TYPE APCControlDI :
STRUCT
	P1ZeroOffsetOutRangeAlm_b	:	BOOL	;
	P1ZeroAdjOutRangeAlm_b	:	BOOL	;
	P1SpanAdjOutRangeAlm_b	:	BOOL	;
	P2ZeroOffsetOutRangeAlm_b	:	BOOL	;
	P2ZeroAdjOutRangeAlm_b	:	BOOL	;
	P2SpanAdjOutRangeAlm_b	:	BOOL	;
	P1PressCtrlInterlockAlm_b	:	BOOL	;
	P2PressCtrlInterlockAlm_b	:	BOOL	;
	ValveOpenCtrlInterlockAlm_b	:	BOOL	;
	ValveHoldCtrlInterlockAlm_b	:	BOOL	;
	ValveCloseInterlockAlm_b	:	BOOL	;
	AutoTeachingInterlockAlm_b	:	BOOL	;
	P1DisconnectionAlm_b	:	BOOL	;
	P2DisconnectionAlm_b	:	BOOL	;
	PumpStopInterlockAlm_b	:	BOOL	;
	AutoTeachingErr1Alm_b	:	BOOL	;
	AutoTeachingErr2Alm_b	:	BOOL	;
	Spare1_b	:	BOOL	;
	Spare2_b	:	BOOL	;
	Spare3_b	:	BOOL	;
	Spare4_b	:	BOOL	;
	Spare5_b	:	BOOL	;
	Spare6_b	:	BOOL	;
	Spare7_b	:	BOOL	;
	Spare8_b	:	BOOL	;
	Spare9_b	:	BOOL	;
	SpareA_b	:	BOOL	;
	SpareB_b	:	BOOL	;
	SpareC_b	:	BOOL	;
	SpareD_b	:	BOOL	;
	SpareE_b	:	BOOL	;
	SpareF_b	:	BOOL	;

END_STRUCT
END_TYPE
